(* Logix 5000 Routine export DeviceNetRouter; software revision 19.01 *)

TYPE AparianDNTRInput :
STRUCT
   Instance : STRING;
   Status : AparianDNTRStatus;
   MappedItemStatus : BOOL[128];
   TransactionRate : DINT;
   Temperature : REAL;
   DeviceNetRxCount : DINT;
   DeviceNetTxCount : DINT;
   DeviceNetCRCError : DINT;
   DeviceNetBitError : DINT;
   DeviceNetStuffError : DINT;
   DeviceNetUCMMOpenCount : DINT;
   DeviceNetUCMMCloseCount : DINT;
   DeviceNetIOConnections : DINT;
   DeviceNetPollCommandCount : DINT;
   DeviceNetFragmentAckErrors : DINT;
   DeviceNetExplicitFragmentErrors : DINT;
   DeviceNetPollFragmentErrors : DINT;
   DeviceNetExplicitClientNotFound : DINT;
   DeviceNetDuplicateNode : DINT;
   TagReads : DINT;
   TagWrites : DINT;
   TagConnectionErrors : DINT;
   TagErrors : DINT;
END_STRUCT
END_TYPE

TYPE AparianDNTRStatus :
STRUCT
   PLCEmulationMode : BOOL;
   ScheduledParameterMode : BOOL;
   ConfigurationValid : BOOL;
END_STRUCT
END_TYPE

VAR_GLOBAL   (* controller tags *)
   DNTR01Input : AparianDNTRInput;
END_VAR

PROGRAM MainProgram

ROUTINE DeviceNetRouter   (* ladder *)
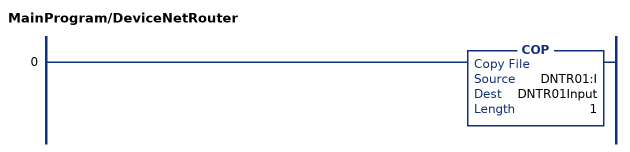
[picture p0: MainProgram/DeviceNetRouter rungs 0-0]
   0: COP(DNTR01:I,DNTR01Input,1);
END_ROUTINE
END_PROGRAM
